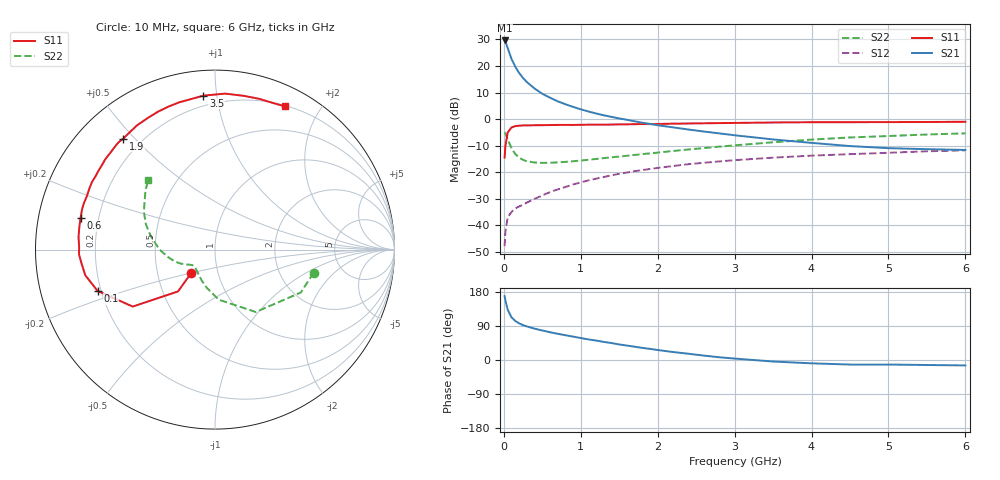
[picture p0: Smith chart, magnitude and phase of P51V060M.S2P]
! SIEMENS Small Signal Semiconductors
! BFP183
! Si NPN RF Bipolar Junction Transistor in SOT143
! VCE = 1 V  IC = 60 mA
! Common Emitter S-Parameters:  March  1996
# GHz  S  MA  R  50
!  f  S11  S21  S12  S22
! GHz  MAG  ANG  MAG  ANG  MAG  ANG  MAG  ANG
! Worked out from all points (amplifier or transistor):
!   36 points, 10 MHz to 6 GHz, reference 50 ohm
!   highest |S21| = 29.6 dB at 10 MHz (marker M1)
!   |S21| within 3 dB of that: start of sweep to 51.78 MHz
!   unconditionally stable (mu >= 1): start of sweep to 40.76 MHz; 111.4 MHz to end of sweep
!   at 250 MHz: K = 1.48, MAG = 19.8 dB, |S12| = -32.3 dB
!   at 1.4 GHz: K = 2.04, MAG = 5.2 dB, |S12| = -21.2 dB
!   at 6 GHz: K = 1.58, MAG = -4.4 dB, |S12| = -11.8 dB
!   S11 on the Smith chart (normalised r, x): 10 MHz: 0.74, -0.20; 100 MHz: 0.19, -0.17; 600 MHz: 0.13, +0.11; 1.9 GHz: 0.13, +0.46; 3.5 GHz: 0.14, +0.92; 6 GHz: 0.21, +1.58
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0.01  0.1878 -135.4  30.33 168.4  0.004 59.0  0.5639 -13.2
0.02  0.3113 -131.5  28.96 157.4  0.0074 60.4  0.5349 -26.5
0.05  0.5575 -145.3  21.84 132.7  0.014 51.4  0.4153 -56.9
0.1  0.6933 -160.6  13.55 112.6  0.0177 40.5  0.2802 -85.6
0.15  0.7368 -168.8  9.616 102.8  0.0207 40.2  0.2175 -102.2
0.2  0.7474 -174.0  7.345 96.6  0.0225 43.0  0.1871 -113.3
0.25  0.7582 -178.0  5.934 92.0  0.0242 44.5  0.1698 -121.1
0.3  0.757 179.2  4.973 88.6  0.0266 48.2  0.16 -127.3
0.4  0.7637 174.6  3.754 82.7  0.0312 52.3  0.1513 -134.6
0.5  0.7662 170.6  2.995 77.9  0.0362 54.7  0.1487 -139.4
0.6  0.7693 166.8  2.524 73.3  0.0419 57.3  0.1496 -142.8
0.7  0.7739 163.2  2.157 69.2  0.047 58.5  0.1521 -145.0
0.8  0.7749 160.4  1.901 65.4  0.0522 59.5  0.1555 -146.4
1.1  0.7821 151.2  1.385 54.3  0.0697 59.4  0.1704 -150.7
1.5  0.7922 140.4  1.026 41.0  0.0925 56.6  0.1959 -155.9
1.9  0.8021 129.6  0.808 29.3  0.1144 52.3  0.2248 -162.2
2.2  0.8173 122.1  0.696 21.0  0.13 48.9  0.2496 -167.6
2.8  0.838 108.0  0.536 7.2  0.1586 41.2  0.3014 -178.7
3.5  0.8602 94.3  0.412 -4.0  0.1869 32.6  0.3643 168.5
4.5  0.8717 79.2  0.309 -12.0  0.2175 20.8  0.4489 152.0
5.5  0.8783 68.5  0.27 -13.2  0.2464 10.8  0.5103 139.4
6  0.8883 63.9  0.261 -14.3  0.2566 5.4  0.537 133.7
